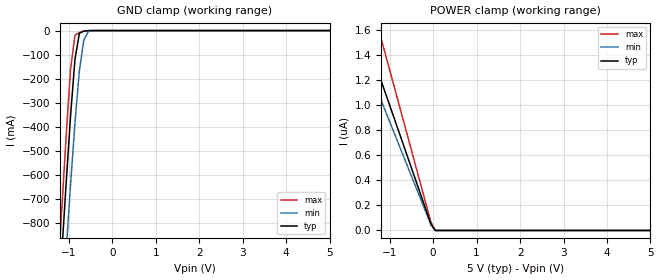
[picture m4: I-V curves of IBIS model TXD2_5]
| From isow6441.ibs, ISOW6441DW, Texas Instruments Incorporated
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|   TXD2_5 Model
[Model]   TXD2_5
Model_type Input
Polarity   Inverting
Enable   Active-High
Vinl =  1.500V
Vinh =  3.500V
C_comp   1.300pF   1.100pF   1.500pF
[Model Spec]
Vinh   3.500V   3.150V   3.850V
Vinl   1.500V   1.350V   1.650V
[Temperature Range]   27.000   0.150k   -55.000
[Voltage Range]   5.000V   4.500V   5.500V
[POWER Clamp Reference]   5.000V   4.500V   5.500V
[GND Clamp Reference]   0.0V   0.0V   0.0V
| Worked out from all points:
|   GND clamp passes 1 mA (typ) near -0.60 V on its own axis
[GND_clamp]
|Voltage   I(typ)   I(min)   I(max)
-5V       -9.981A    -9.605A    -10.39A
-1.263V   -1.228A    -1.489A    -1.058A
-1.162V   -926.2mA   -1.199A    -742.2mA
-1.061V   -632.1mA   -914.7mA   -437mA
-960mV    -354.1mA   -640.4mA   -159.5mA
-859mV    -119.1mA   -384.3mA   -19.49mA
-758mV    -11.66mA   -168mA     -8.159mA
-657mV    -1.816mA   -40.64mA   -2.858mA
-556mV    -292.6uA   -4.614mA   -391.8uA
-455mV    -21.33uA   -343.7uA   -16.09uA
5V        0A         0A         -639.7nA
[POWER_clamp]
|Voltage   I(typ)   I(min)   I(max)
-5V       4.989uA    4.333uA    6.397uA
-1.868V   1.864uA    1.619uA    2.39uA
-1.767V   1.763uA    1.532uA    2.261uA
-1.666V   1.662uA    1.444uA    2.132uA
-1.565V   1.562uA    1.357uA    2.002uA
-1.262V   1.259uA    1.095uA    1.615uA
-1.161V   1.159uA    1.007uA    1.486uA
-50mV     49.95nA    45.12nA    64.04nA
51mV      0A         0A         0A
5V        0A         0A         0A
